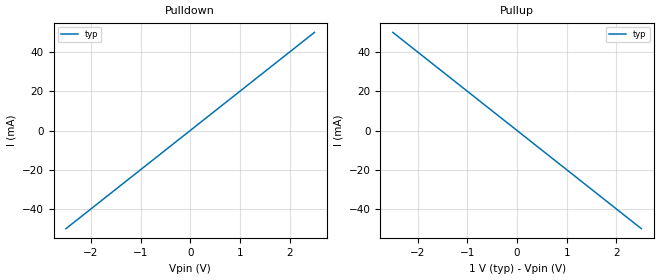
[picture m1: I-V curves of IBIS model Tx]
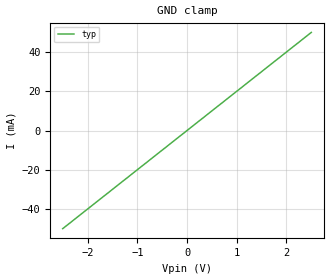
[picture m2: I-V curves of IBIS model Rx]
[IBIS Ver]   3.2
[Disclaimer] THIS IBIS MODEL HAS BEEN CREATED BY  SIGNAL
   INTEGRITY SOFTWARE
[File Name]  incremental.ibs
[File Rev]   1.0
[Date]   Tue Aug 28 14:09:44 EDT 2012
[Source]   Signal Integrity Software
   6 Clock Tower Place, Suite 250
   Maynard, MA 01754
   support@sisoft.com
   Auto-generated by "Create Default Model" dialog.
[Notes]   Note
[Copyright]  No Copyright
[Component]  incremental
[Manufacturer]  SiSoft
[Package]
R_pkg 0.001m   NA   NA
L_pkg 0.001nH  NA   NA
C_pkg 0.001pF  NA   NA
[Pin]  signal_name   model_name   R_pin  L_pin  C_pin
AW10 RX[0]_N Rx NA NA NA
AV10 RX[0]_P Rx NA NA NA
AW13 RX[1]_N Rx NA NA NA
AV13 RX[1]_P Rx NA NA NA
AW8 RX[10]_N Rx NA NA NA
AV8 RX[10]_P Rx NA NA NA
AR10 TX[0]_N Tx NA NA NA
AP10 TX[0]_P Tx NA NA NA
AR13 TX[1]_N Tx NA NA NA
AP13 TX[1]_P Tx NA NA NA
AR8 TX[10]_N Tx NA NA NA
AP8 TX[10]_P Tx NA NA NA
[Diff_Pin]  inv_pin  vdiff  tdelay_typ  tdelay_min  tdelay_max
AV10   AW10   0.1V   0.0ns   0.0ns   0.0ns
AV13   AW13   0.1V   0.0ns   0.0ns   0.0ns
AV8   AW8   0.1V   0.0ns   0.0ns   0.0ns
AP10   AR10   0.1V   0.0ns   0.0ns   0.0ns
AP13   AR13   0.1V   0.0ns   0.0ns   0.0ns
AP8   AR8   0.1V   0.0ns   0.0ns   0.0ns
| Models and submodels in the file (2): Tx (Output), Rx (Input)
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|   MODEL Tx
[Model] Tx
Model_type Output
C_comp 0p NA NA
Cref = 0
Vref = 0.5
Rref = 50
Vmeas = 0.5
[Temperature_Range] 25 100 0
[Voltage Range] 1.0 0.9 1.1
[Tstonefile] Tx_typ.s4p Tx_min.s4p Tx_max.s4p
|[Tstonefile] ami_file.ami(Tstonefile)
[Tstonefile Ports] Buffer+ Buffer- Pad+ Pad-
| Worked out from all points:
|   slope of the pulldown table from 0 to 0.15 V, typ, clamps not added: 50 ohm
|   slope of the pullup table from 0 to 0.15 V, typ, clamps not added: 50 ohm
[Pulldown]
-2.5V     -50mA      NA         NA
0V        0A         NA         NA
2.5V      50mA       NA         NA
[Pullup]
-2.5V     50mA       NA         NA
0V        0A         NA         NA
2.5V      -50mA      NA         NA
[Ramp]
dV/dt_r .3/60p .27/1p .33/1p
dV/dt_f .3/60p .27/1p .33/1p
|   MODEL Rx
[Model] Rx
Model_type Input
C_comp 0.0p NA NA
Vinh = 0.55
Vinl = 0.45
[Temperature_Range] 25 100 0
[Voltage Range] 1.0 0.9 1.1
[Tstonefile] Rx_typ.s4p Rx_min.s4p Rx_max.s4p
|[Tstonefile] ami_file.ami(Tstonefile)
[Tstonefile Ports] Pad+ Pad- Buffer+ Buffer-
[GND Clamp]
-2.5V     -50mA      NA         NA
0V        0A         NA         NA
2.5V      50mA       NA         NA
[Pin_Package_IBIS-ISS]
  AW10 Pkg Length=0.01755
  AV10 Pkg Length=0.01755
  AW13 Pkg Length=0.01565
  AV13 Pkg Length=0.01565
  AW8  Pkg Length=0.01785
  AV8  Pkg Length=0.01785
  AR10 Pkg Length=0.01375
  AP10 Pkg Length=0.01375
  AR13 Pkg Length=0.01165
  AP13 Pkg Length=0.01165
  AR8  Pkg Length=0.01340
  AP8  Pkg Length=0.01340
[End_Pin_Package_IBIS-ISS]
[Model_Package_IBIS-ISS]
  Tx Pkg L=0.02
  Rx Pkg L=0.01
  Tx Pkg_Coupled Length=0.02
  Rx Pkg_Coupled Length=0.01
[End_Model_Package_IBIS-ISS]
[Package_IBIS-ISS]
  [Package] Pkg
   File typ pkg_typ.mod
   Subckt typ pkg_typ
   Type Differential
   [Parameters]
   Length 0.02
   [End_Parameters]
   [Model_Ports]
   1 PadP
   2 PadM
   3 PinP
   4 PinM
   [End_Model_Ports]
  [End_Package]
  [Package] Pkg_Coupled
   File pkg_coupled_{Corner}.mod
   Subckt pkg_coupled_{Corner}
   Type Coupled_Differential
   [Parameters]
   Length 0.02
   [End_Parameters]
   [Model_Ports]
   1 PadP
   2 PadM
   3 PinP
   4 PinM
   5 PadA1P
   6 PadA1M
   7 PinA1P
   8 PinA1M
   9 PadA2P
   10 PadA2M
   11 PinA2P
   12 PinA2M
   [End_Model_Ports]
  [End_Package]
[End_Package_IBIS-ISS]
